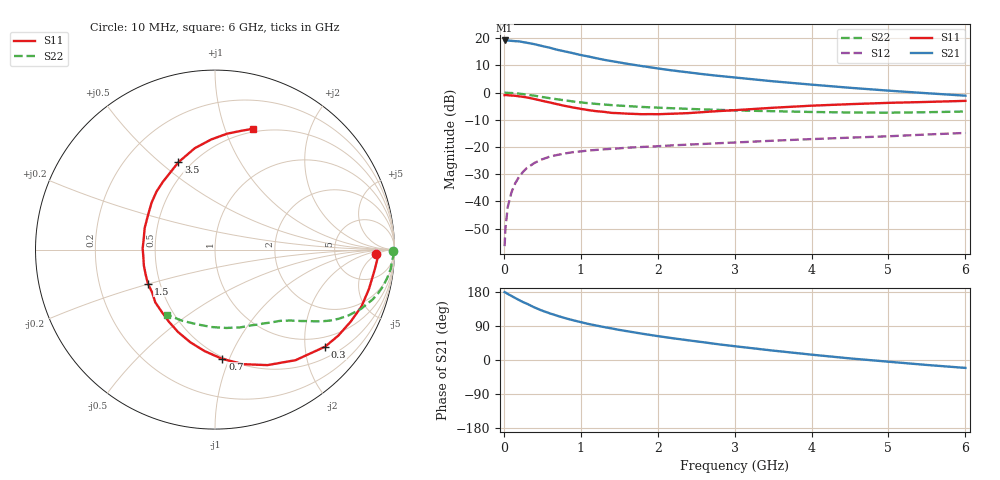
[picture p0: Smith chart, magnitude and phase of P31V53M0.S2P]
! SIEMENS Small Signal Semiconductors
! BFP181
! Si NPN RF Bipolar Junction Transistor in SOT143
! VCE = 1.5 V  IC = 3 mA
! Common Emitter S-Parameters:  March  1996
# GHz  S  MA  R  50
!  f  S11  S21  S12  S22
! GHz  MAG  ANG  MAG  ANG  MAG  ANG  MAG  ANG
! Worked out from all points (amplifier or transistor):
!   36 points, 10 MHz to 6 GHz, reference 50 ohm
!   highest |S21| = 19.2 dB at 10 MHz (marker M1)
!   |S21| within 3 dB of that: start of sweep to 639.1 MHz
!   unconditionally stable (mu >= 1): 1.974 GHz to end of sweep
!   at 250 MHz: K = 0.17, MSG = 23.9 dB, |S12| = -29.1 dB
!   at 1.4 GHz: K = 0.79, MSG = 16.1 dB, |S12| = -20.7 dB
!   at 6 GHz: K = 1.10, MAG = 4.9 dB, |S12| = -14.8 dB
!   S11 on the Smith chart (normalised r, x): 10 MHz: 17, -4; 300 MHz: 0.75, -2.45; 700 MHz: 0.49, -0.94; 1.5 GHz: 0.43, -0.20; 3.5 GHz: 0.43, +0.58; 6 GHz: 0.47, +1.25
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0.01  0.8977 -1.6  9.123 179.0  0.0015 84.8  0.9933 -0.6
0.02  0.9069 -3.1  9.088 178.3  0.0031 84.3  0.9977 -1.3
0.05  0.8971 -7.0  9.103 174.4  0.0078 87.2  0.99 -3.2
0.1  0.8855 -14.3  8.969 169.0  0.0148 80.0  0.9847 -6.3
0.2  0.8558 -28.0  8.77 158.0  0.0286 73.9  0.9582 -12.3
0.25  0.8374 -35.0  8.511 152.7  0.035 69.8  0.9402 -15.1
0.3  0.8178 -41.4  8.273 148.5  0.0412 66.9  0.9208 -17.6
0.4  0.7624 -53.9  7.782 138.5  0.0512 60.8  0.8778 -22.1
0.5  0.7067 -65.6  7.196 130.1  0.0595 55.0  0.8313 -26.1
0.6  0.658 -76.0  6.688 122.9  0.0668 50.6  0.7898 -29.2
0.7  0.6108 -86.1  6.117 116.4  0.0717 47.0  0.7526 -31.7
0.9  0.5344 -104.9  5.318 104.9  0.0804 41.0  0.6888 -35.5
1.1  0.4774 -122.4  4.624 95.1  0.0863 36.9  0.6395 -38.5
1.3  0.444 -138.5  4.029 87.0  0.0907 33.9  0.6048 -41.0
1.5  0.419 -153.2  3.6 79.4  0.0945 32.0  0.5772 -43.2
1.8  0.4012 -174.6  3.073 69.3  0.1003 30.1  0.5456 -46.6
2.2  0.41 162.7  2.552 57.3  0.1073 27.9  0.5164 -51.6
2.8  0.4591 135.2  2.03 41.2  0.1177 25.6  0.4823 -60.1
3.5  0.5275 112.8  1.617 24.8  0.1307 22.8  0.456 -71.8
4.5  0.6143 91.9  1.229 4.2  0.1487 18.4  0.4318 -92.7
5.5  0.675 78.1  0.976 -13.1  0.1699 14.4  0.4369 -115.0
6  0.7062 72.5  0.88 -20.9  0.1816 11.4  0.4497 -126.3
